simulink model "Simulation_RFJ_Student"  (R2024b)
settings: Solver=ode23  StartTime=0.0  StopTime=10.0  MaxStep=1e-1  RelTol=1e-3  EnableMultiTasking=on

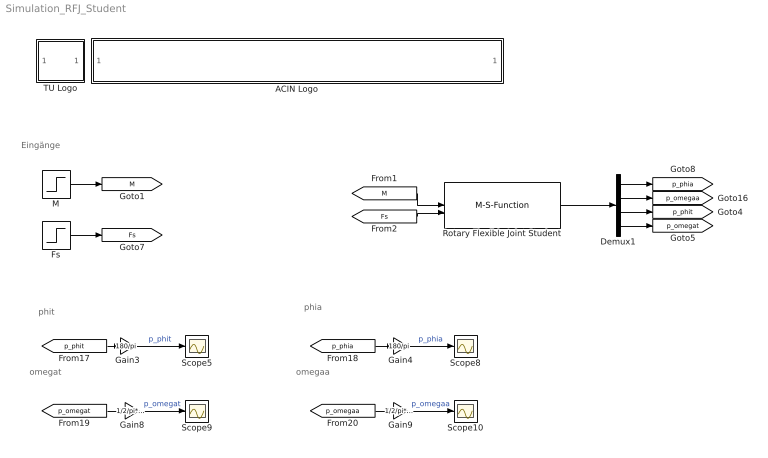
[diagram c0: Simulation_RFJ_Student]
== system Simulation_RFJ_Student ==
  note: Eingänge
  note: phit
  note: phia
  note: omegat
  note: omegaa
  ACIN Logo : Subsystem
      mask init:
      | s = get_param(gcb,'UserData');
  Demux1 : Demux
  Fs : Step  Time=5  After=0  SampleTime=0
  Gain3 : Gain  Gain=180/pi
  Gain4 : Gain  Gain=180/pi
  Gain8 : Gain  Gain=1/2/pi*60
  Gain9 : Gain  Gain=1/2/pi*60
  M : Step  Time=1/10  Before=1/10  After=0  SampleTime=0
  Rotary Flexible Joint Student : M-S-Function  FunctionName=RFJ_Student_S
  Scope{5,8..10} (4 alike) : Scope
  TU Logo : Subsystem
      mask init:
      | s = get_param(gcb,'UserData');
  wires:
  M/1 -> [M]
  Fs/1 -> [Fs]
  Gain3/1 -> Scope5/1  "p_phit"
  Gain4/1 -> Scope8/1  "p_phia"
  Gain8/1 -> Scope9/1  "p_omegat"
  Gain9/1 -> Scope10/1  "p_omegaa"
  [p_phit] -> Gain3/1
  [p_phia] -> Gain4/1
  [p_omegat] -> Gain8/1
  [p_omegaa] -> Gain9/1
  Demux1/1 -> [p_phia]
  Demux1/2 -> [p_omegaa]
  Demux1/3 -> [p_phit]
  Demux1/4 -> [p_omegat]
  [M] -> Rotary Flexible Joint Student/1
  [Fs] -> Rotary Flexible Joint Student/2
  Rotary Flexible Joint Student/1 -> Demux1/1

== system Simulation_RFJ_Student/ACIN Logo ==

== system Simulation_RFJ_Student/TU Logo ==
